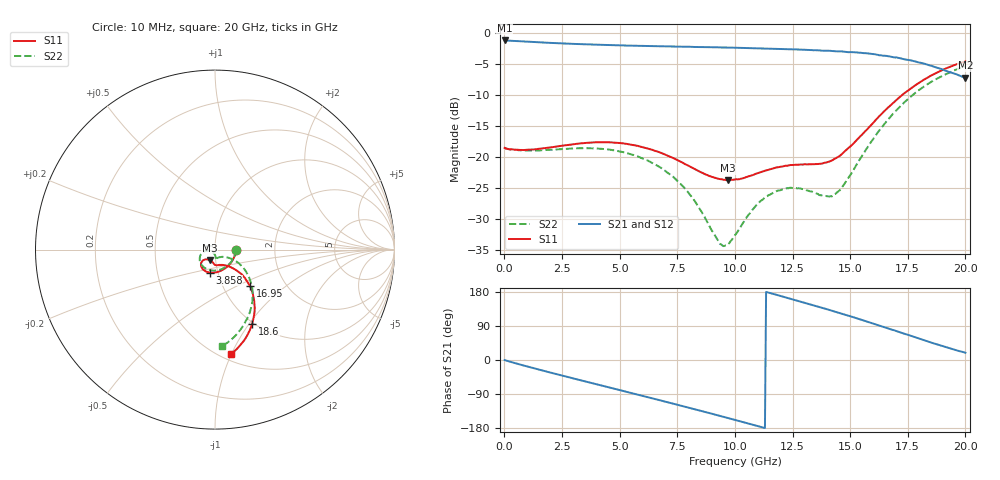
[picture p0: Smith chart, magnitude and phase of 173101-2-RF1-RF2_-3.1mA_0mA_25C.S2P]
!  2-Port S-parameters saved by WinCal
! VAR MeasName=S-Parameters (CALIBRATED_DATA) read from VNA (N5242A)
! VAR MeasDate=2017-7-20 9:33:11
! VAR NAME=173101-2-RF1-RF2_-3.1mA_0mA_25C
! VAR FILENAME=173101-2-RF1-RF2_-3.1mA_0mA_25C.S2P
! VAR DATE=2017-7-20 9:33:11
! VAR PHYS_PORTS=1,2
# Hz S DB R 50
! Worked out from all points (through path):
!   401 points, 10 MHz to 20 GHz, reference 50 ohm
!   highest |S21| = -1.19 dB at 10 MHz (marker M1); lowest = -7.2 dB at 20 GHz (marker M2)
!   group delay of S21, straight-line fit = 46.7 ps
!   lowest |S11| = -23.7 dB at 9.705 GHz (marker M3), VSWR 1.14, Z = 46.8 - j5.46 ohm
!   |S11| at or under -10 dB: start of sweep to 17.25 GHz
!   |S22| runs from -34.3 to -5.3 dB; largest |S21 - S12| = 0.0066
!   S11 on the Smith chart (normalised r, x): 10 MHz: 1.27, -0.00; 3.858 GHz: 0.91, -0.24; 16.95 GHz: 1.33, -0.59; 18.6 GHz: 0.98, -1.04; 20 GHz: 0.55, -0.99
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1e7  -18.51 -0.8  -1.19 -0.2  -1.19 -0.2  -18.46 -0.8
1.50925e9  -18.65 -53.4  -1.49 -25.5  -1.49 -25.5  -18.92 -55.7
3.358325e9  -17.76 -94.8  -1.80 -54.2  -1.80 -54.2  -18.55 -103.3
3.858075e9  -17.63 -103.1  -1.86 -61.9  -1.86 -61.8  -18.57 -113.5
5.357325e9  -17.90 -123.3  -2.01 -84.8  -2.03 -84.7  -19.40 -140.7
6.70665e9  -19.18 -135.3  -2.12 -105.7  -2.11 -105.6  -21.52 -160.6
8.055975e9  -21.53 -137.2  -2.21 -126.8  -2.23 -126.7  -26.08 -172.6
9.355325e9  -23.54 -122.7  -2.32 -147.6  -2.30 -147.5  -33.99 -141.4
9.70515e9  -23.74 -116.8  -2.33 -153.2  -2.33 -153.2  -34.06 -117.6
1.0005e10  -23.60 -111.5  -2.37 -158.1  -2.37 -158.1  -32.57 -100.4
1.085458e10  -22.77 -99.2  -2.44 -172.0  -2.44 -171.9  -28.09 -84.6
1.155422e10  -21.93 -94.0  -2.50 176.2  -2.51 176.4  -25.97 -85.6
1.235382e10  -21.32 -89.6  -2.60 162.7  -2.61 162.8  -24.96 -87.8
1.335332e10  -21.14 -80.9  -2.74 145.4  -2.72 145.6  -25.57 -84.5
1.410295e10  -20.70 -67.2  -2.85 132.0  -2.87 132.1  -26.34 -66.2
1.450275e10  -19.89 -58.8  -2.96 124.8  -2.96 125.0  -25.46 -50.4
1.570215e10  -15.66 -44.0  -3.26 101.9  -3.28 102.2  -18.71 -28.6
1.670165e10  -11.83 -45.0  -3.76 82.2  -3.79 82.2  -13.71 -34.7
1.695152e10  -10.97 -46.3  -3.94 77.4  -3.93 77.5  -12.64 -37.9
1.78011e10  -8.48 -54.2  -4.54 60.2  -4.54 60.3  -9.72 -50.1
1.86007e10  -6.67 -63.5  -5.39 44.4  -5.41 44.6  -7.69 -63.1
2e10  -4.58 -81.5  -7.19 19.1  -7.24 19.8  -5.34 -86.0
